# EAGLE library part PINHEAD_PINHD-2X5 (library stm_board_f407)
PIN HEADER
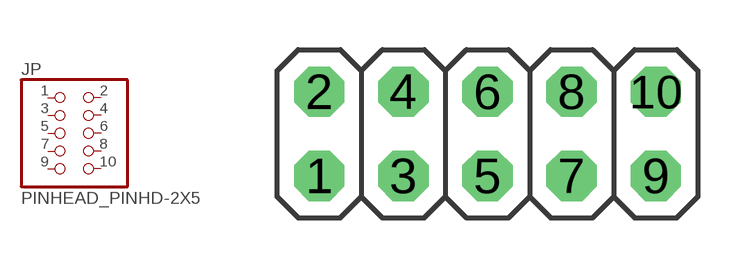
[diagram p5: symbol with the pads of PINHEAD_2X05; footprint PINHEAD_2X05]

Designator prefix JP

## PINHEAD_PINHD-2X5  [PINHEAD_2X05]
1  1  pas
2  2  pas
3  3  pas
4  4  pas
5  5  pas
6  6  pas
7  7  pas
8  8  pas
9  9  pas
10  10  pas

## Footprint PINHEAD_2X05 (pad centres in mm)
PIN HEADER
drill 1.016 octagon: 1 -5.08,-1.27; 2 -5.08,1.27; 3 -2.54,-1.27; 4 -2.54,1.27; 5 0,-1.27; 6 0,1.27; 7 2.54,-1.27; 8 2.54,1.27; 9 5.08,-1.27; 10 5.08,1.27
